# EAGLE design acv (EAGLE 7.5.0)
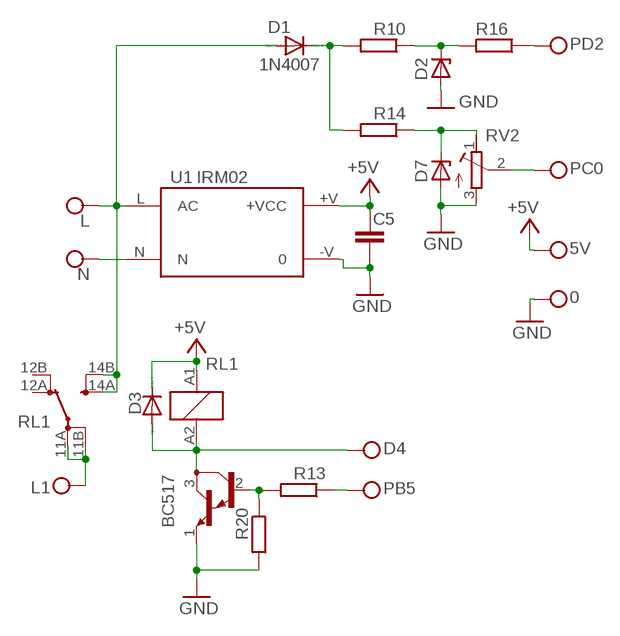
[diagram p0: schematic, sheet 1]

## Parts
0  CONNWIRE  [CONNWIRE]
5V  CONNWIRE  [CONNWIRE]
C5  C-EUC1206  [C1206]
D1  1N4007  1N4004  [DO41-10]
D2  1N4733  ZPY  [DO41Z10]
D3  1N4004  [DO41-10]
D4  CONNWIRE  [CONNWIRE]
D7  1N4733  ZPY  [DO41Z10]
L  CONNWIRE  [CONNWIRE]
L1  CONNWIRE  [CONNWIRE]
N  CONNWIRE  [CONNWIRE]
PB5  CONNWIRE  [CONNWIRE]
PC0  CONNWIRE  [CONNWIRE]
PD2  CONNWIRE  [CONNWIRE]
Q1  BC517  [TO92]
R10  R-EU_V235/17  [V235/17]
R13  R-EU_M1206  [M1206]
R14  R-EU_V235/17  [V235/17]
R16  R-EU_M1206  [M1206]
R20  R-EU_M1206  [M1206]
RL1  RZ03-1A4-D005  RTH14012  [RT-C/O16A5]
RV2  R-TRIMM-3386-F  [R-TRIMM-3386F]
U1  IRM02  [IRM02]

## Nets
+5V: 5V.P$1 C5.1 D3.C RL1.A1 U1.+V(+VCC)
GND: 0.P$1 C5.2 D2.A D7.A Q1.1(E) R20.2 RV2.3(E) U1.-V
N$1: D1.A L.P$1 RL1.14A(2:SA) RL1.14B(2:SB) U1.L(AC)
N$2: N.P$1 U1.N
N$3: D1.C R10.2 R14.2
N$4: D2.C R10.1 R16.2
N$5: D7.C R14.1 RV2.1(A)
N$10: PD2.P$1 R16.1
N$25: PC0.P$1 RV2.2(S)
N$28: Q1.2(B) R13.2 R20.1
N$29: D3.A D4.P$1 Q1.3(C) RL1.A2
N$30: L1.P$1 RL1.11A(2:PA) RL1.11B(2:PB)
N$31: PB5.P$1 R13.1
Unconnected: RL1.12A(2:OA) RL1.12B(2:OB)

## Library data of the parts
0 5V D4 L L1 N PB5 PC0 PD2 = connholes:CONNWIRE
C5 = rcl:C-EU: CAPACITOR, European symbol
D1 D3 = diode:1N4004: DIODE
D2 D7 = diode:ZPY: Z DIODE
Q1 = transistor-npn:BC517*: NPN Darlington Transistor
R10 R13 R14 R16 R20 = resistor:R-EU_: RESISTOR, European symbol
RL1 = relay:RTH14*: Power PCB Relay 105°C 16A SCHRACK 1 pole 16 A, high-temperature version Source: http://www.schrack.com/.. 5831.pdf; MPN: RTH14012; OC_FARNELL: 1629018; OC_NEWARK: 03P2408
RV2 = rcl:R-TRIMM-3386-F
U1 = acdc:IRM02: 2W Single Output ACDC converter

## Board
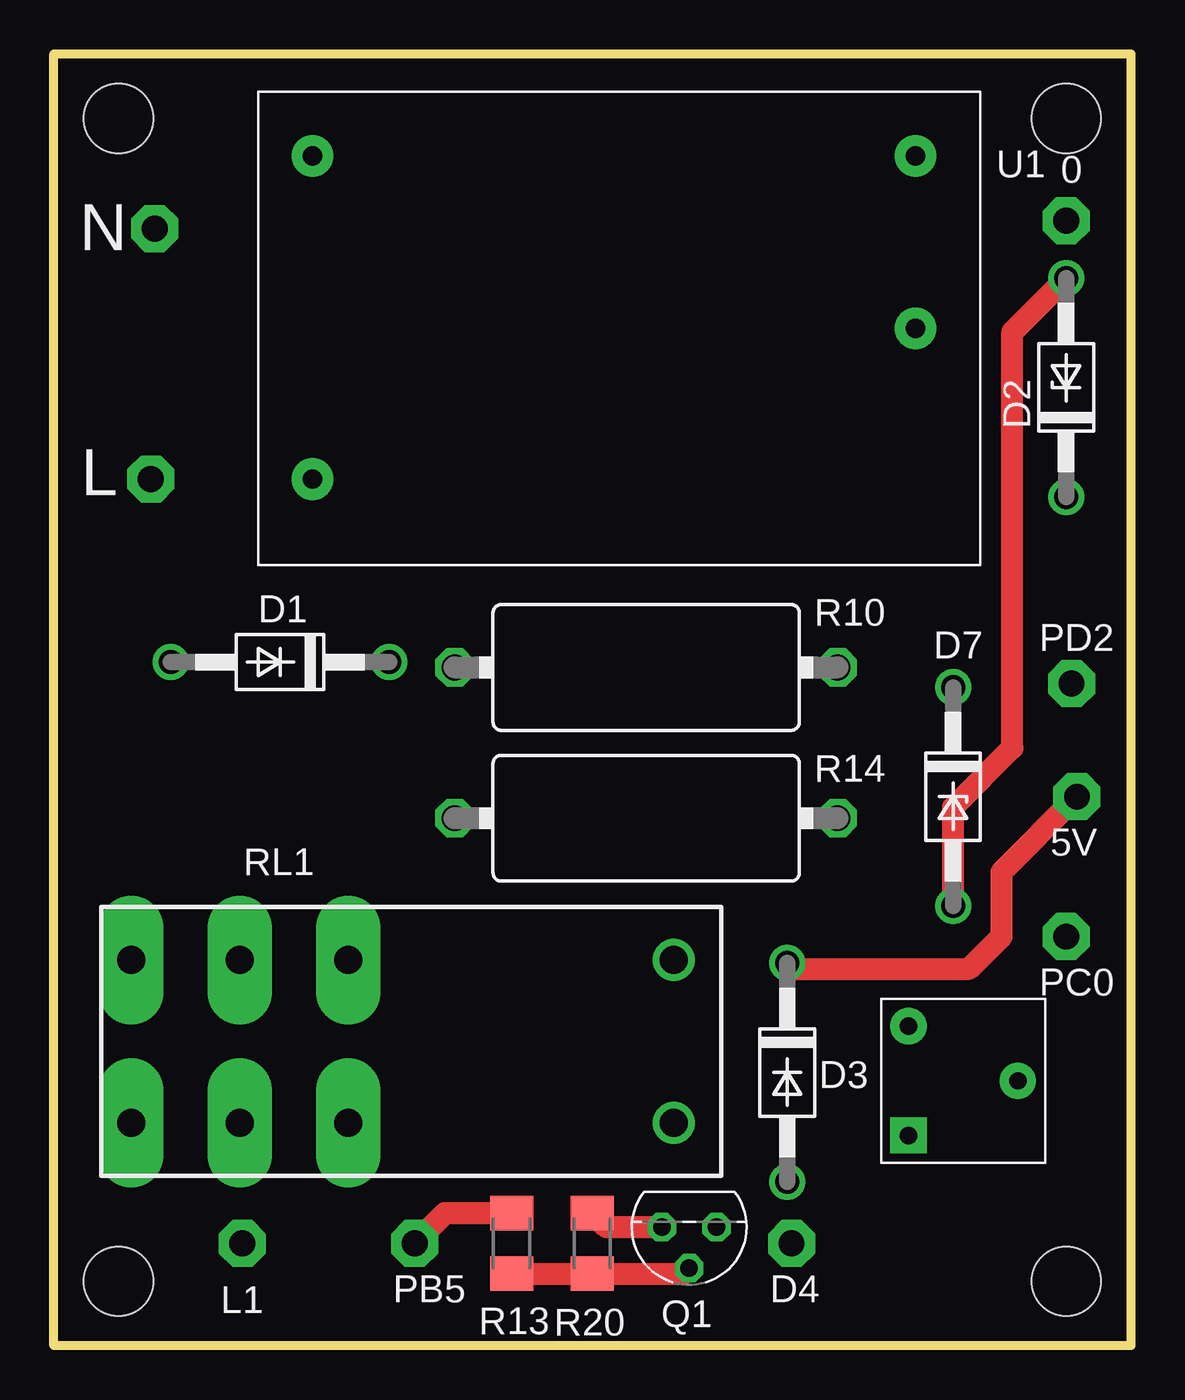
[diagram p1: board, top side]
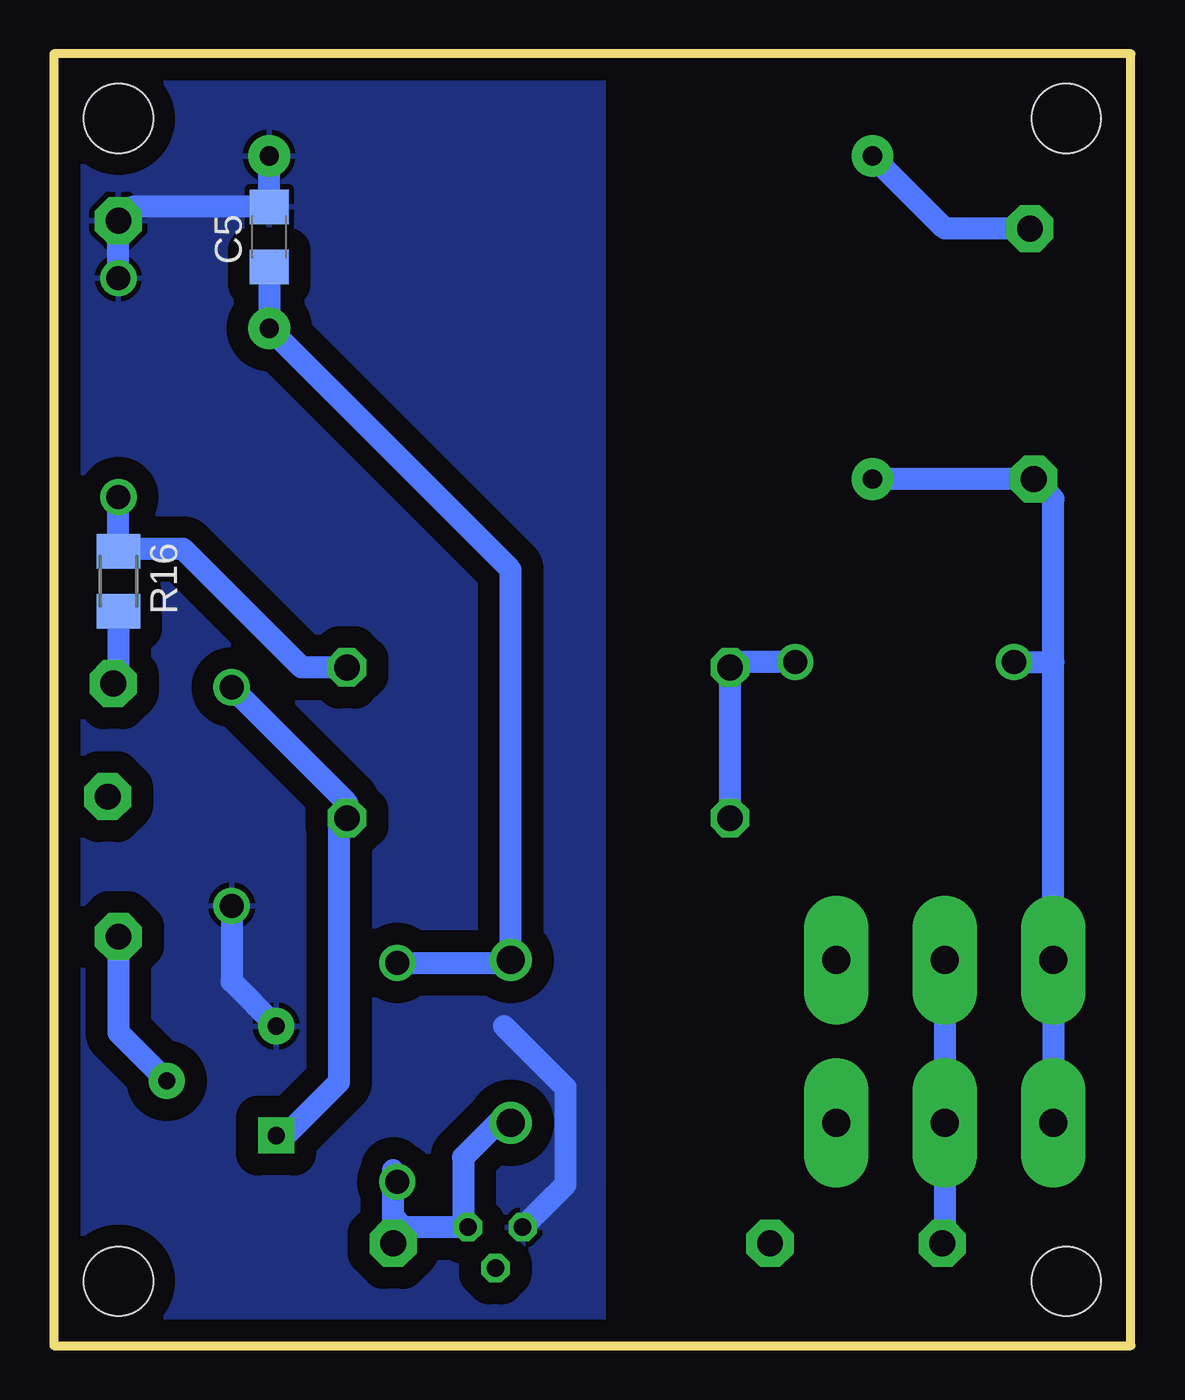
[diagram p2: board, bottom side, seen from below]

Size 50 x 60 mm. Coordinates in mm from the lower left corner, seen from the top.
Outline: 0,0 0,60 50,60 50,0 0,0
Copper layers (1*16): Top 0.035mm / dielectric 1.5mm / Bottom 0.035mm
Design rules "default": minimum track width 10mil, minimum drill 24mil, track to track 8mil, track to pad 8mil, pad to pad 8mil, via to via 8mil, smd to smd 8mil, copper to edge 40mil, drill to drill 8mil, minimum pad ring 10mil, minimum via ring 8mil, stop-mask expansion 4mil, vias tented up to drill 0mil, thermal gap 10mil
Holes 3.2 mm at 3,57 47,57 3,3 47,3

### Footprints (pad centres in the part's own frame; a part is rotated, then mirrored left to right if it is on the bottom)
CONNWIRE = drill 1.2 pad 2.184 octagon: P$1 0,0
C1206 = smd 1.6 x 1.8: 1 -1.4,0; 2 1.4,0
DO41-10 = drill 1.118: A 5.08,0; C -5.08,0
DO41Z10 = drill 1.118: A 5.08,0; C -5.08,0
TO92 = drill 0.813 octagon: 1 1.27,0; 2 0,1.905; 3 -1.27,0
V235/17 = drill 1.194 octagon: 1 -8.89,0; 2 8.89,0
M1206 = smd 1.6 x 2: 1 -1.4,0; 2 1.4,0
RT-C/O16A5 = drill 1.3 pad 3 long: 11A 7.56,3.78; 11B 7.56,-3.78; 12A 2.52,3.78; 12B 2.52,-3.78; 14A 12.6,3.78; 14B 12.6,-3.78 | drill 1.3: A1 -12.6,-3.78; A2 -12.6,3.78
R-TRIMM-3386F = drill 0.8 pad 1.676 square: 1 0,0 | drill 0.8 pad 1.676: 2 5.08,2.54; 3 0,5.08
IRM02 = drill 0.9 pad 1.93: +V 30.5,-11; -V 30.5,-3; L 2.5,-18; N 2.5,-3

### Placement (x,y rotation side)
0  47,52.25 0 top
5V  47.5,25.5 0 top
C5  40,51.5 90 bottom
D1  10.5,31.75 180 top
D2  47,44.5 90 top
D3  34.05,12.69 270 top
D4  34.25,4.75 0 top
D7  41.75,25.5 270 top
L  4.5,40.25 0 top
L1  8.75,4.75 0 top
N  4.68,51.88 0 top
PB5  16.75,4.75 0 top
PC0  47,19 0 top
PD2  47.25,30.75 0 top
Q1  29.5,5.5 180 top
R10  27.5,31.5 180 top
R13  21.25,4.75 270 top
R14  27.5,24.5 180 top
R16  47,35.5 90 bottom
R20  25,4.75 90 top
RL1  16.19,14.13 180 top
RV2  39.68,9.76 0 top
U1  9.5,58.25 0 top

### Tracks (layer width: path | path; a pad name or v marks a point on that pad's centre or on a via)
+5V
  Top 1.016: D3.C 34.32,17.5 42.5,17.5 44,19 44,22 5V.P$1
  Bottom 1.016: C5.1 U1.+V 28.79,36.04 RL1.A1 28.93,17.77 D3.C
GND
  Top 1.016: D7.A 41.75,25 44.5,27.75 44.5,47.08 D2.A | Q1.1 25.65,5.5 R20.2
  Bottom 1.016: U1.-V C5.2 46.35,52.9 0.P$1 D2.A | D7.A 41.75,16.91 RV2.3 | 29.09,14.84 26.25,12 26.25,7.48 Q1.1
  pour Bottom (isolate 1.016): 24.75,59 49.25,59 49.25,0.75 24.5,0.75 24.5,41 24.5,59
N$1
  Bottom 1.016: U1.L L.P$1 3.59,39.34 3.59,31.75 | 3.59,31.75 RL1.14B RL1.14A | D1.A 3.59,31.75
N$2
  Bottom 1.016: N.P$1 8.63,51.88 U1.N
N$3
  Bottom 1.016: D1.C 18.36,31.75 R10.2 R14.2
N$4
  Bottom 1.016: R10.1 38.5,31.5 44,37 46.9,37 R16.2 D2.C
N$5
  Bottom 1.016: RV2.1 39.24,9.76 36.75,12.25 36.75,24.14 R14.1 36.39,25.22 D7.C
N$10
  Bottom 1.016: R16.1 47,31 PD2.P$1
N$25
  Bottom 1.016: PC0.P$1 47,14.54 RV2.2
N$28
  Top 1.016: R13.2 R20.1 29.25,3.35 Q1.2
N$29
  Bottom 1.016: D4.P$1 34.25,6 | 34.25,6 34.25,8.16 D3.A | 34.25,6 33.75,5.5 Q1.3 31,5.73 31,8.75 29.4,10.35 RL1.A2
N$30
  Bottom 1.016: RL1.11B RL1.11A 8.63,4.87 L1.P$1
N$31
  Top 1.016: R13.1 18.15,6.15 PB5.P$1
